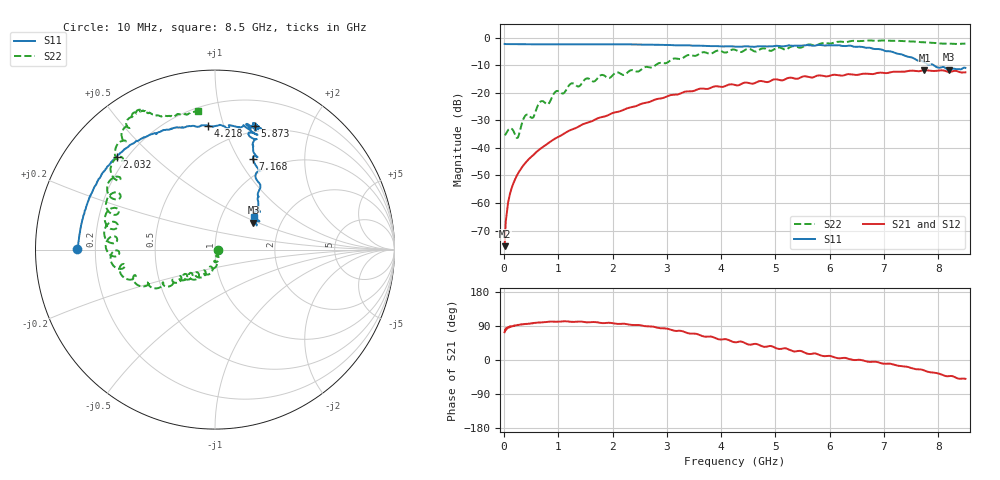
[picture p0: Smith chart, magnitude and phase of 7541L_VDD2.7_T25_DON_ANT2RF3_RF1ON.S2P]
!Agilent Technologies,E5071C,MY46417908,A.11.23
!Date: Wed Dec 09 17:17:19 2020
!Data & Calibration Information:
!Freq	S11:SOLT2(ON)	S21:SOLT2(ON)	S12:SOLT2(ON)	S22:SOLT2(ON)
!PortZ  Port1:50+j0  Port2:50+j0
!Above PortZ is port z conversion or system Z0 setting when saving the data.
!When reading, reference impedance value at option line is always used.
# Hz S dB R 50
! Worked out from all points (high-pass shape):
!   1601 points, 10 MHz to 8.5 GHz, reference 50 ohm
!   highest |S21| = -11.82 dB at 7.747 GHz (marker M1); lowest = -75.6 dB at 10 MHz (marker M2)
!   |S21| within 3 dB of the highest: 5.207 GHz to 5.347 GHz (140.6 MHz wide, 2.66 % of centre); 5.423 GHz to end of sweep
!   lowest |S11| = -11.6 dB at 8.192 GHz (marker M3), VSWR 1.71, Z = 72.8 + j23.5 ohm
!   |S11| at or under -10 dB: 7.916 GHz to end of sweep
!   |S22| runs from -36.4 to -1.0 dB; largest |S21 - S12| = 0.0025
!   S11 on the Smith chart (normalised r, x): 10 MHz: 0.13, +0.00; 2.032 GHz: 0.16, +0.39; 4.218 GHz: 0.33, +0.88; 5.873 GHz: 0.44, +1.27; 7.168 GHz: 0.80, +1.15; 8.5 GHz: 1.42, +0.56
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1e7  -2.30 179.6  -75.63 73.4  -75.27 75.4  -35.37 -3.5
6.836875e7  -2.35 178.3  -60.64 85.1  -60.66 85.3  -33.73 -21.5
1.16125e8  -2.36 177.2  -56.20 88.2  -56.13 87.9  -32.88 -41.5
2.43475e8  -2.39 174.3  -49.76 92.5  -49.78 92.4  -36.34 -55.1
3.230688e8  -2.40 172.4  -47.22 93.6  -47.27 94.1  -31.51 -44.5
4.026625e8  -2.40 170.7  -45.18 95.1  -45.23 95.2  -28.10 -67.2
5.353188e8  -2.41 167.7  -42.62 96.9  -42.60 96.9  -28.96 -72.2
6.732812e8  -2.43 164.7  -40.26 99.1  -40.24 99.2  -23.21 -80.5
8.059375e8  -2.42 161.8  -38.43 100.7  -38.44 100.9  -24.16 -89.2
9.598188e8  -2.42 158.1  -36.38 101.0  -36.40 100.9  -19.44 -95.9
1.426769e9  -2.41 148.6  -31.68 101.3  -31.68 101.2  -16.76 -111.3
2.031681e9  -2.46 136.7  -27.16 96.1  -27.15 96.1  -13.04 -131.5
2.843538e9  -2.61 123.0  -22.17 84.7  -22.18 84.7  -9.33 -143.1
4.217856e9  -3.19 93.5  -17.00 47.7  -17.01 47.8  -4.31 178.4
4.255e9  -3.26 91.9  -17.18 46.8  -17.18 46.8  -4.40 175.1
5.671769e9  -2.90 70.3  -14.48 16.5  -14.43 16.3  -2.60 135.7
5.873406e9  -2.82 72.2  -13.85 10.6  -13.79 10.9  -1.96 133.2
7.088538e9  -4.91 66.3  -12.73 -9.6  -12.78 -9.6  -1.13 118.1
7.168131e9  -5.25 67.2  -12.40 -11.7  -12.41 -11.6  -1.15 118.5
7.746512e9  -8.99 47.3  -11.82 -28.0  -11.83 -28.0  -1.70 114.0
8.192238e9  -11.64 35.0  -12.44 -42.7  -12.48 -42.6  -2.15 104.8
8.5e9  -10.97 40.0  -12.59 -49.6  -12.67 -49.4  -2.17 96.8
